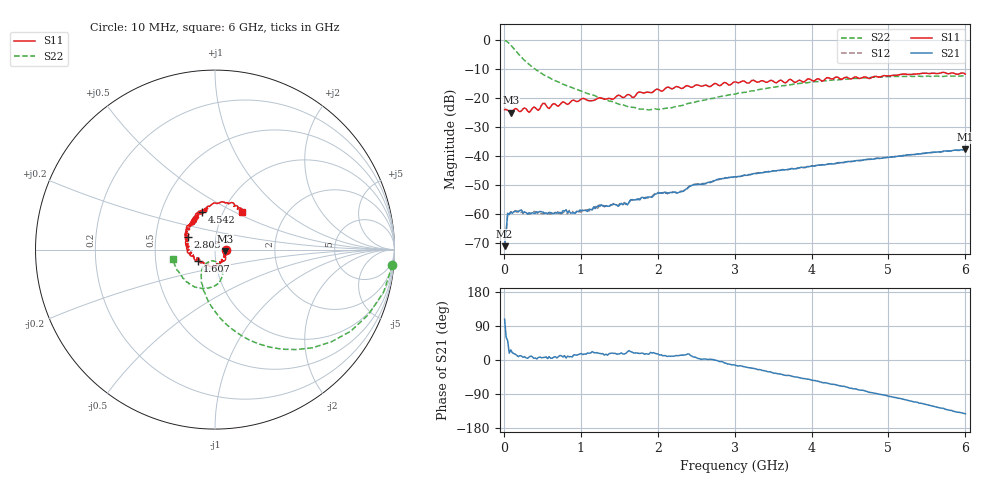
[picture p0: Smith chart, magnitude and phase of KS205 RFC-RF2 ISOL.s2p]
!Agilent	"Technologies,E5071B,JP1KK00126,A.08.11"
!Date:	Wed	Mar	27	12:09:53	2013
!Data	&	Calibration	Information:
!Freq	S11:SOLT2(ON)	S21:SOLT2(ON)	S12:SOLT2(ON)	S22:SOLT2(ON)
#	Hz	S	dB	R	50
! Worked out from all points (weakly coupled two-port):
!   301 points, 10 MHz to 6 GHz, reference 50 ohm
!   highest |S21| = -37.70 dB at 6 GHz (marker M1); lowest = -71.2 dB at 10 MHz (marker M2)
!   lowest |S11| = -25.0 dB at 89.87 MHz (marker M3), VSWR 1.12, Z = 55.9 - j1.02 ohm
!   |S11| at or under -10 dB: start of sweep to end of sweep
!   |S22| runs from -24.1 to -0.1 dB; largest |S21 - S12| = 0.00022
!   S11 on the Smith chart (normalised r, x): 10 MHz: 1.13, -0.00; 1.607 GHz: 0.82, -0.10; 2.805 GHz: 0.73, +0.10; 4.542 GHz: 0.79, +0.35; 6 GHz: 1.22, +0.55
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1e7  -24.00 -1.5  -71.20 108.0  -70.70 108.0  -0.07 -5.0
2.996667e7  -23.90 -4.4  -66.00 60.3  -66.80 59.8  -0.28 -14.1
4.993333e7  -24.20 -8.3  -59.80 51.0  -59.90 55.0  -0.64 -22.9
8.986667e7  -25.00 -9.3  -59.40 26.7  -59.30 28.7  -1.65 -38.4
1.897e8  -24.40 -20.2  -59.30 8.8  -59.10 8.7  -4.74 -65.1
2.695667e8  -23.40 -24.2  -59.40 9.1  -59.30 6.1  -6.96 -78.3
3.294667e8  -24.90 -29.0  -59.60 7.7  -60.10 5.5  -8.37 -85.8
3.893667e8  -23.10 -33.2  -59.80 4.4  -59.20 6.3  -9.65 -91.9
4.492667e8  -24.20 -37.9  -59.50 6.9  -60.10 3.9  -10.70 -97.2
5.091667e8  -21.80 -44.0  -59.40 6.5  -60.00 5.7  -11.80 -102.0
5.890333e8  -23.60 -55.6  -59.50 8.8  -60.00 10.3  -12.90 -107.0
1.0283e9  -20.10 -105.0  -58.90 14.3  -58.40 13.8  -17.80 -123.0
1.607333e9  -18.80 -148.0  -56.90 21.6  -56.50 17.8  -22.90 -115.0
1.6872e9  -19.80 -151.0  -55.20 18.4  -55.20 18.4  -23.20 -111.0
2.006667e9  -17.00 -172.0  -52.60 15.6  -52.90 13.2  -23.90 -92.6
2.246267e9  -16.00 177.0  -52.90 11.7  -52.70 12.5  -22.80 -81.8
2.805333e9  -15.70 155.0  -47.90 -4.3  -48.10 -4.0  -19.50 -69.3
3.005e9  -14.40 149.0  -47.20 -13.7  -47.20 -13.1  -18.60 -69.1
4.0233e9  -14.10 121.0  -43.50 -54.0  -43.50 -53.9  -14.40 -85.1
4.542433e9  -13.00 109.0  -41.80 -76.1  -41.90 -75.5  -13.20 -100.0
5.001667e9  -12.30 96.9  -40.50 -95.7  -40.40 -95.6  -12.60 -116.0
6e9  -11.70 54.2  -37.70 -142.0  -37.80 -142.0  -12.30 -167.0
